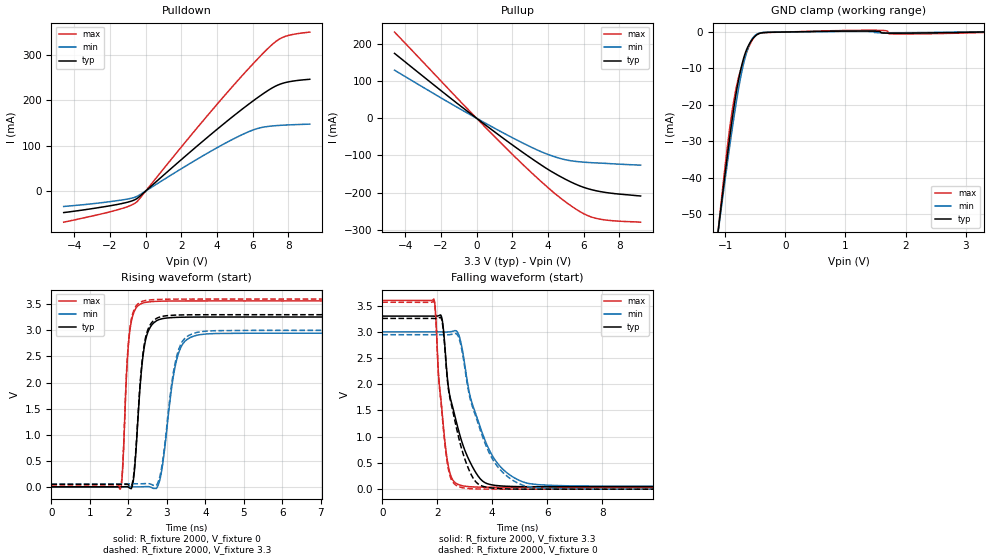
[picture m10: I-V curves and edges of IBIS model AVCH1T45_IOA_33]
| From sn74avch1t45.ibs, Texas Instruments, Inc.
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[Model]   AVCH1T45_IOA_33
Model_type  I/O
Vinl=0.8
Vinh=2.0
Enable   Active-Low
Vref =   0
Rref =   2000
Cref =   15p
Vmeas =   1.65
| variable   typ   min   max
C_comp   4.94pF   3.95pF   5.92pF
| C_pullup   3.99pF   3.00pF   5.23pF
| C_pulldown   4.19pF   3.63pF   4.72pF
| C_tri-state   4.94pF   3.95pF   5.92pF
[Temperature Range]   40   100   -40
| Ambient temperature   25   85   -40
[Voltage range]   3.3   3   3.6
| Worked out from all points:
|   slope of the pulldown table from 0 to 0.495 V, typ, clamps not added: 28.7 ohm
|   slope of the pullup table from 0 to 0.495 V, typ, clamps not added: 27.4 ohm
|   GND clamp passes 1 mA (typ) near -0.49 V on its own axis
|   rising waveform, R_fixture 2000, V_fixture 0: 20-80 % time 204ps typ, 310ps min, 142ps max; typ from 0 V to 3.26 V
|   falling waveform, R_fixture 2000, V_fixture 3.3: 20-80 % time 750ps typ, 1.01ns min, 331ps max; typ from 3.3 V to 0.046 V
|   rising waveform, R_fixture 2000, V_fixture 3.3: 20-80 % time 203ps typ, 308ps min, 142ps max; typ from 0.046 V to 3.3 V
|   falling waveform, R_fixture 2000, V_fixture 0: 20-80 % time 666ps typ, 1.01ns min, 326ps max; typ from 3.26 V to 0 V
[GND Clamp]
| AVCH1T45_IOA_33
|   Voltage   I(typ)   I(min)   I(max)
-4.6V     -599.7mA   -548.3mA   -664.9mA
-1.12V    -55.23mA   -55.37mA   -55.14mA
-1.09V    -51.05mA   -51.59mA   -50.43mA
-920mV    -28.51mA   -30.95mA   -25.9mA
-800mV    -15.23mA   -17.87mA   -14.13mA
-710mV    -8.287mA   -9.958mA   -8.772mA
-615mV    -3.828mA   -4.226mA   -4.458mA
-540mV    -1.856mA   -1.633mA   -1.986mA
-430mV    -403.7uA   -315.6uA   -401.2uA
1.325V    252.6uA    143.2uA    467.7uA
1.81V     -334.6uA   -204.5uA   -541uA
3.3V      1.645nA    73.67uA    -145.7uA
[Pulldown]
| AVCH1T45_IOA_33
|   Voltage   I(typ)   I(min)   I(max)
-4.6V     -47.48mA   -33.99mA   -68.59mA
-1.68V    -30.25mA   -21.7mA    -42.42mA
-975mV    -24.15mA   -17.32mA   -33.81mA
-545mV    -17.86mA   -12.84mA   -25.24mA
2.535V    87.18mA    61.73mA    122.4mA
4.495V    151.5mA    105.8mA    213.1mA
5.9V      194.5mA    132.3mA    274.6mA
6.8V      219.5mA    141.6mA    311.3mA
7.31V     231.1mA    143.7mA    329.1mA
7.725V    237.2mA    144.7mA    338.4mA
8.275V    241.7mA    145.7mA    344.4mA
9.2V      245.6mA    146.9mA    349.3mA
[Pullup]
| AVCH1T45_IOA_33
|   Voltage   I(typ)   I(min)   I(max)
-4.6V     174.2mA    129.1mA    231.4mA
-1.105V   40.58mA    29.86mA    54.82mA
1.575V    -56.66mA   -41.45mA   -76.65mA
3.53V     -122.6mA   -88.07mA   -166.1mA
4.725V    -157.4mA   -108.5mA   -215.1mA
5.775V    -181.6mA   -117mA     -250.3mA
6.525V    -192.9mA   -119.7mA   -266.7mA
7.455V    -200.9mA   -121.9mA   -274.6mA
9.2V      -209mA     -126mA     -279.3mA
[Ramp]
| AVCH1T45_IOA_33
| variable   typ   min   max
dV/dt_r   1.98/2.07E-10   1.79/3.16E-10   2.17/1.45E-10
dV/dt_f   1.97/7.50E-10   1.78/1.01E-09   2.15/3.32E-10
R_load = 2000
[Rising Waveform]
| AVCH1T45_IOA_33
R_fixture =   2000
C_fixture =   0
L_fixture =   0
V_fixture =   0
V_fixture_min = 0
V_fixture_max = 0
|   Time   V(typ)   V(min)   V(max)
0s        37.78nV    120nV      1.948nV
1.795ns   -44.04uV   -5.702uV   -34.44mV
2.045ns   -28.74mV   28.53uV    3.035V
2.145ns   225.9mV    27.83uV    3.35V
2.335ns   2.201V     141.4uV    3.513V
2.475ns   2.898V     4.051mV    3.54V
2.825ns   3.213V     160.8mV    3.559V
3.31ns    3.25V      2.579V     3.564V
3.88ns    3.255V     2.92V      3.564V
29.99ns   3.256V     2.946V     3.564V
[Falling Waveform]
| AVCH1T45_IOA_33
R_fixture =   2000
C_fixture =   0
L_fixture =   0
V_fixture =   3.3
V_fixture_min = 3
V_fixture_max = 3.6
|   Time   V(typ)   V(min)   V(max)
0s        3.3V       3V         3.6V
1.88ns    3.299V     3V         3.62V
2.055ns   3.308V     3V         2.134V
2.17ns    3.261V     2.999V     1.517V
2.36ns    2.183V     2.996V     579.6mV
2.9ns     899.4mV    2.701V     67.04mV
3.22ns    491.4mV    1.726V     45.54mV
3.895ns   93.22mV    747.2mV    36.97mV
5.35ns    47.14mV    105.8mV    35.99mV
29.99ns   46.09mV    58.43mV    35.95mV
[Rising Waveform]
| AVCH1T45_IOA_33
R_fixture =   2000
C_fixture =   0
L_fixture =   0
V_fixture =   3.3
V_fixture_min = 3
V_fixture_max = 3.6
|   Time   V(typ)   V(min)   V(max)
0s        46.09mV    58.43mV    35.95mV
1.795ns   46.05mV    58.42mV    1.389mV
2.045ns   17.23mV    58.46mV    3.075V
2.145ns   273.2mV    58.46mV    3.391V
2.335ns   2.253V     58.57mV    3.549V
2.47ns    2.935V     62.4mV     3.575V
2.825ns   3.258V     221.5mV    3.595V
3.305ns   3.294V     2.633V     3.599V
3.875ns   3.299V     2.973V     3.6V
29.99ns   3.3V       3V         3.6V
[Falling Waveform]
| AVCH1T45_IOA_33
R_fixture =   2000
C_fixture =   0
L_fixture =   0
V_fixture =   0
V_fixture_min = 0
V_fixture_max = 0
|   Time   V(typ)   V(min)   V(max)
0s        3.256V     2.946V     3.564V
1.88ns    3.255V     2.946V     3.585V
2.17ns    3.217V     2.945V     1.475V
2.355ns   2.172V     2.942V     543.1mV
2.54ns    1.56V      2.953V     158.7mV
2.89ns    768.2mV    2.673V     31.45mV
3.215ns   300.6mV    1.691V     9.403mV
3.885ns   28.88mV    700.1mV    1.01mV
5.31ns    665.9uV    48.27mV    36.52uV
29.99ns   553.7nV    810.5nV    233.7nV
